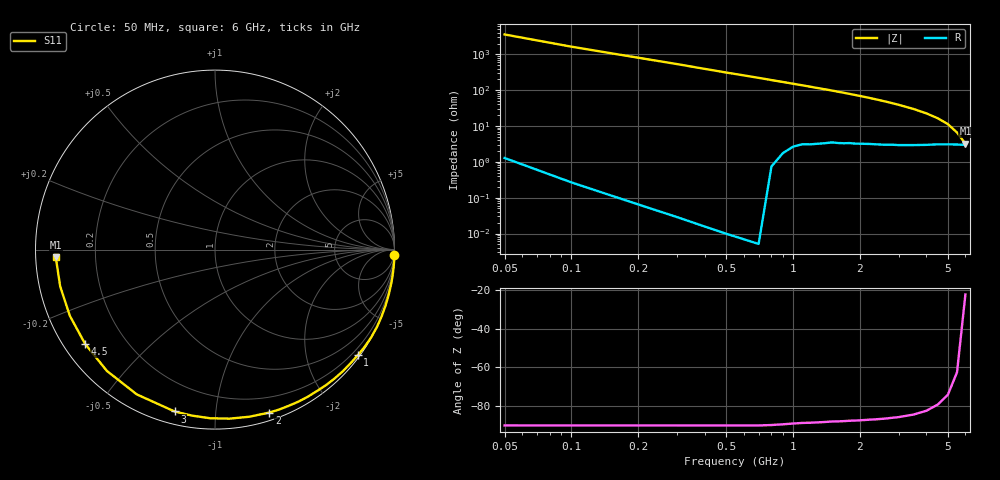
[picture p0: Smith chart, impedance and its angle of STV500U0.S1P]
! SIEMENS Discrete & RF Semiconductors
! BA892
! Si PIN Diode in SCD-80
! VR = 0.5 V
! S-Parameters:  September  1997
# GHz  S  MA  R  50
!  f  S11
! GHz  MAG  ANG
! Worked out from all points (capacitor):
!   34 points, 50 MHz to 6 GHz, reference 50 ohm
!   read as one part to ground: C = 973 fF near 50 MHz
!   lowest |Z| = 3.21 ohm at 6 GHz (marker M1)
!   S11 on the Smith chart (normalised r, x): 50 MHz: 0, -72; 1 GHz: 0.05, -3.03; 2 GHz: 0.06, -1.38; 3 GHz: 0.06, -0.78; 4.5 GHz: 0.06, -0.32; 6 GHz: 0.06, -0.02
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0.05  1 -1.6
0.25  1 -8.9
0.4  1 -14.5
0.5  1 -18.3
0.6  1 -21.9
0.7  1 -25.5
0.8  0.9981 -29.3
0.9  0.9944 -32.9
1  0.9897 -36.5
1.2  0.9831 -43.7
1.3  0.9796 -47.3
1.4  0.9758 -50.8
1.5  0.9714 -54.2
1.6  0.969 -57.9
1.8  0.9623 -64.8
1.9  0.9601 -68.2
2  0.957 -71.6
2.2  0.9507 -78.4
2.4  0.9452 -85.1
2.6  0.9401 -91.6
2.8  0.9338 -97.9
3  0.9296 -104.0
3.5  0.9169 -118.4
4  0.9054 -131.7
4.5  0.8943 -144.0
5  0.8888 -155.4
5.5  0.8866 -166.6
6  0.888 -177.2
